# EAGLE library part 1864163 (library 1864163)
PCB direct plug, nominal cross section: 2.5 mm?, color: green, nominal current: 12 A, rated voltage (III/2): 320 V, contact surface: Tin, Number of potentials: 15, Number of rows: 1, Number of positions per row: 15, number of connections: 15, product range: SDC 2,5/..-PV, pitch: 5 mm, connection method: Push-in spring connection, mounting: SKEDD - Direct plug-in technology, conductor/PCB connection direction: 90 ?, pin layout: Zigzag pinning W, solder pin [P]: 4.7 mm, Stecksystem: SKEDD, Locking: Snap-in lo Source: Datasheet
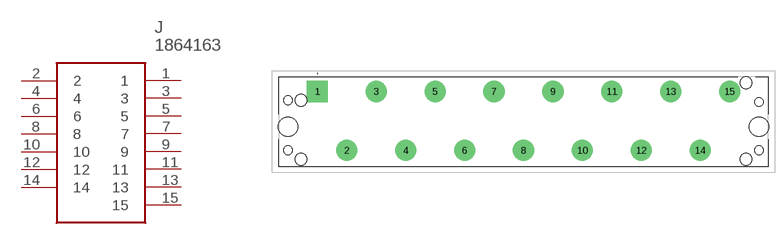
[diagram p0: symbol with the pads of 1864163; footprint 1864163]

Designator prefix J

## 1864163 (Description: PCB direct plug, nominal cross section: 2.5 mm?, color: green, nominal current: 12 A, rated voltage (III/2): 320 V, contact surface: Tin, Number of potentials: 15, Number of rows: 1, Number of positions per row: 15, number of connections: 15, product range: SDC 2,5/..-PV, pitch: 5 mm, connection method: Push-in spring connection, mounting: SKEDD - Direct plug-in technology, conductor/PCB connection direction: 90 ?, pin layout: Zigzag pinning W, solder pin [P]: 4.7 mm, Stecksystem: SKEDD, Locking: Snap-in lo; Height: 16.35mm; Manufacturer_Name: Phoenix Contact; Manufacturer_Part_Number: 1864163; Mouser_Part_Number: 651-1864163; Mouser_Price-Stock: https://www.mouser.com/Search/Refine.aspx?Keyword=651-1864163)  [1864163]
1  1
2  2
3  3
4  4
5  5
6  6
7  7
8  8
9  9
10  10
11  11
12  12
13  13
14  14
15  15

## Footprint 1864163 (pad centres in mm)
1864163
drill 2.4 pad 3.6 square: 1 0,0
drill 2.4 pad 3.6: 2 5,-10; 3 10,0; 4 15,-10; 5 20,0; 6 25,-10; 7 30,0; 8 35,-10; 9 40,0; 10 45,-10; 11 50,0; 12 55,-10; 13 60,0; 14 65,-10; 15 70,0
hole 3.3 at -5,-6
hole 3.3 at 75,-6
hole 2 at -2.8,-11.5
hole 2 at -2.8,-1.5
hole 2 at 72.8,-11.5
hole 2 at 72.8,1.5
hole 1.5 at -5,-10
hole 1.5 at -5,-1.5
hole 1.5 at 75,-10
hole 1.5 at 75,-1.8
